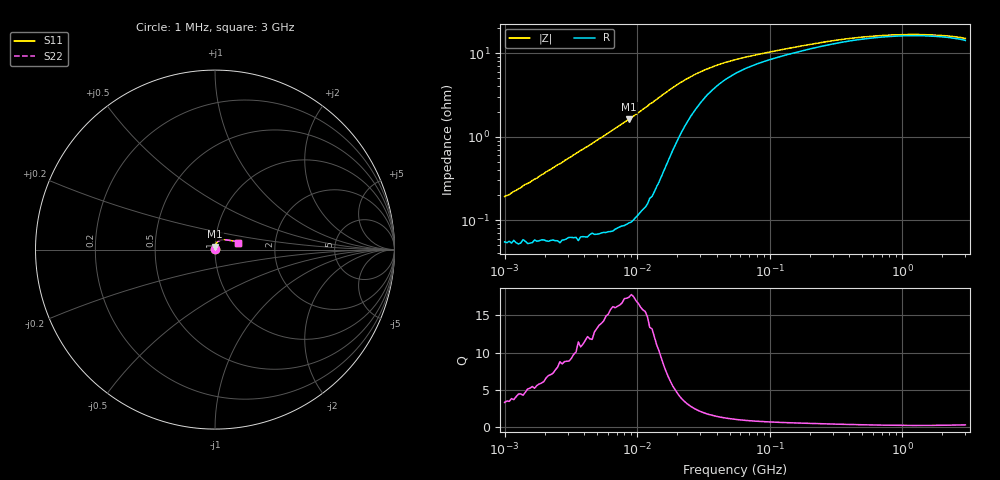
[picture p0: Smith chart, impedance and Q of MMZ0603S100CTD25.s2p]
! S-parameter Generated by TDK Corporation
! Copyright(C) 2018 TDK Corporation.
! All Rights Reserved.
! TDK P/N: MMZ0603S100CTD25 (Chip Bead)
! Property: |Z|=10¶ at 100MHz
! Size(LxWxT): 0.6x0.3x0.3mm, 0.024x0.012x0.012inches
! Model Type: s2p (Touchstone File Format Version 1.0)
! Frequency: DC=Yes Start=1MHz Stop=3000MHz 202points Log-sweep
! Model Generated on Aug. 6, 2018
! Port Assignments:
!  1 ---@@@--- 2
! Applicable Conditions:
!  Temperature = 25 degC
!  DC Bias Current = 0 A
!  Small Signal Operation
! Terms and conditions regarding TDK Simulation Models
! (1)This simulation model is being provided solely for informational purposes. Please refer to the specifications of the products in terms of detailed characteristics of such products.
! (2)In no event shall TDK Corporation of any of its subsidiaries be liable for any loss or damage arising, directly or indirectly,
!  From any information contained in this simulation model, including, but not limited to loss or damages arising from any inaccuracies, omissions or errors in connection with such information.
! (3)Any and all copyrights on this simulation model are owned by TDK Corporation.
!  Duplication or redistribution of this simulation model without prior written permission from TDK Corporation is prohibited.
! (4)This simulation model is subject to any modification or change without any prior notice.
! (5)Neither TDK Corporation nor any of its subsidiaries shall make any warranty, express or implied,
!  Including but not limited to the correctness, implied warranties of merchantability and fitness for a particular purpose with respect to this simulation models.
! (6)The use of this simulation model shall be deemed to have consented to the terms and conditions hereof.
# Hz S MA R 50
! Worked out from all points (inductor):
!   201 points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, 1 MHz to 3 GHz, reference 50 ohm
!   read as one part in series: L = 29 nH near 1.041 MHz
!   highest Q = 17.4 at 8.686 MHz (marker M1), where L = 29.7 nH
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1000000  0.001921 73.3  0.9994 -0.1  0.9994 -0.1  0.001921 73.3
1083356  0.002027 73.9  0.9994 -0.1  0.9994 -0.1  0.002027 73.9
1433740  0.002686 77.8  0.9994 -0.2  0.9994 -0.2  0.002686 77.8
1553251  0.002841 79.0  0.9995 -0.2  0.9995 -0.2  0.002841 79.0
1616692  0.002994 79.5  0.9995 -0.2  0.9995 -0.2  0.002994 79.5
1751453  0.00319 79.7  0.9994 -0.2  0.9994 -0.2  0.00319 79.7
1897447  0.003499 80.2  0.9994 -0.2  0.9994 -0.2  0.003499 80.2
3900413  0.007114 84.5  0.9993 -0.4  0.9993 -0.4  0.007114 84.5
4577760  0.008286 84.7  0.9993 -0.5  0.9993 -0.5  0.008286 84.7
8686058  0.0162 85.8  0.9989 -0.9  0.9989 -0.9  0.0162 85.8
1.461624e7  0.02937 82.8  0.9967 -1.7  0.9967 -1.7  0.02937 82.8
2.095589e7  0.04351 74.0  0.9889 -2.4  0.9889 -2.4  0.04351 74.0
2.773354e7  0.05513 64.6  0.9776 -2.9  0.9776 -2.9  0.05513 64.6
3.820236e7  0.06734 53.8  0.9618 -3.2  0.9618 -3.2  0.06734 53.8
5.477226e7  0.07905 43.8  0.9445 -3.3  0.9445 -3.3  0.07905 43.8
8.507507e7  0.0911 35.1  0.927 -3.2  0.927 -3.2  0.0911 35.1
2.136344e8  0.1161 24.3  0.8954 -3.1  0.8954 -3.1  0.1161 24.3
4.219165e8  0.1329 17.9  0.8745 -2.7  0.8745 -2.7  0.1329 17.9
8.005644e8  0.1423 13.7  0.8623 -2.2  0.8623 -2.2  0.1423 13.7
1.645649e9  0.1431 12.6  0.861 -2.1  0.861 -2.1  0.1431 12.6
2.266846e9  0.1392 14.1  0.8657 -2.2  0.8657 -2.2  0.1392 14.1
3e9  0.1314 16.1  0.8745 -2.4  0.8745 -2.4  0.1314 16.1
